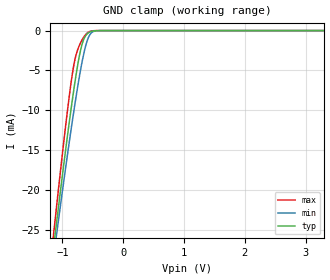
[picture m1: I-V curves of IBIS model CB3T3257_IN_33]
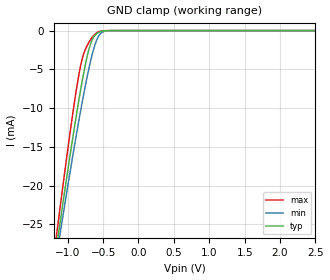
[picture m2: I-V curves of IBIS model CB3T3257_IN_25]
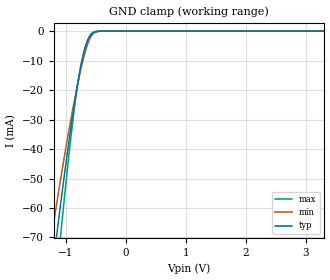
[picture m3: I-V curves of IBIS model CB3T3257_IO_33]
| TEXAS INSTRUMENTS INCORPORATED
| Standard Linear and Logic Group
| IBIS Model of SN74CB3T3257
| 3.3-V LOW-VOLTAGE 4-BIT 1-OF-2 FET MULTIPLEXER/DEMULTIPLEXER WITH 5-V-
| TOLERANT/LEVEL SHIFTER
| This file contains package information for the following:
|  TSSOP 16-pin (PW) package as [Component] CB3T3257_PW
|  TVSOP 16-pin (DGV) package as [Component] CB3T3257_DGV
| This device can be powered at the following Vccs:
|  3.3 volt Vcc
|  2.5 volt Vcc
| This file provides unique models under the [Model Selector] for each Vcc.
| For operation at a specific Vcc, select the appropriate model after each
| [Model Selector] keyword.
[IBIS Ver]   3.2
[Comment char]  |_char
[File Name]   sn74cb3t3257.ibs
[File Rev]   1.1 | a_die
[Date]   August 21, 2003
[Source]   Data created from TI-SPICE simulations at TI-SLL.
[Notes]   The following is an IBIS list for the CB3T3257.
   Please contact sllibis@ti.com with questions and
   comments concerning SLL IBIS models.
   - Non-monotonic data due to FET characteristics.
   - Power clamp data deleted as there is no power-clamp diode.
[Disclaimer] Property of Texas Instruments Incorporated.  Unauthorized
   reproduction and/or distribution is strictly prohibited.
   This product is protected under copyright law.
   Created  2003, (C) Copyright  2003, Texas Instruments
   Incorporated, All Rights Reserved
   UNLESS THERE IS A SIGNED, WRITTEN AGREEMENT TO THE
   CONTRARY, TEXAS INSTRUMENTS (TI) IS PROVIDING THE IBIS
   MODELS  AND WITHOUT ANY WARRANTY, EXPRESSED OR
   IMPLIED.  TI assumes no liability for:
   1) the accuracy of the IBIS models provided to your
   company;
   2) the proper functioning of these IBIS Models in your
   design or for any resulting applications; or
   3) infringement of patents, copyrights or intellectual
   property rights resulting from your use of these IBIS
   models.
   TI provides IBIS Models as a service to our customers.
   You and your company shall not distribute, sell or give
   these models to anyone else without prior written
   permission from TI.
   TI reserves the right to make changes to our products or
   to discontinue any semiconductor product or service
   without notice, and advises our customers to obtain the
   latest version of relevant information to verify, before
   placing orders, that the information being relied on is
   current.
   Please be aware that your receipt and use of the IBIS
   information provided shall serve as acceptance of these
   terms and conditions.  If you do not accept these terms,
   you should return or destroy the IBIS models and any
   other accompanying information immediately.
| Component CB3T3257_PW 16-pin TSSOP
[Component]   CB3T3257_PW
[Manufacturer]   Texas Instruments, Inc.
[Package]
|   typ   min   max
R_pkg   4.500e-02   3.800e-02   5.100e-02
L_pkg   2.593e-09   2.447e-09   3.080e-09
C_pkg   2.810e-13   2.430e-13   3.770e-13
[Pin]   signal_name   model_name   R_pin   L_pin   C_pin
1   S   CB3T3257_IN   4.000e-02   3.080e-09   3.770e-13
2   1B1   CB3T3257_IO   3.800e-02   2.458e-09   2.810e-13
3   1B2   CB3T3257_IO   5.100e-02   2.512e-09   2.550e-13
4   1A   CB3T3257_IO   5.100e-02   2.447e-09   2.430e-13
5   2B1   CB3T3257_IO   5.100e-02   2.447e-09   2.430e-13
6   2B2   CB3T3257_IO   5.100e-02   2.512e-09   2.550e-13
7   2A   CB3T3257_IO   3.800e-02   2.458e-09   2.810e-13
8   GND   GND   4.000e-02   3.080e-09   3.770e-13
9   3A   CB3T3257_IO   3.900e-02   2.832e-09   3.160e-13
10   3B2   CB3T3257_IO   3.800e-02   2.460e-09   2.790e-13
11   3B1   CB3T3257_IO   5.100e-02   2.512e-09   2.550e-13
12   4A   CB3T3257_IO   5.100e-02   2.447e-09   2.430e-13
13   4B2   CB3T3257_IO   5.100e-02   2.447e-09   2.430e-13
14   4B1   CB3T3257_IO   5.100e-02   2.512e-09   2.550e-13
15   NOE   CB3T3257_IN   3.800e-02   2.459e-09   2.790e-13
16   VCC   POWER   3.900e-02   2.832e-09   3.160e-13
| Component CB3T3257_DGV 16-pin TVSOP
[Component]   CB3T3257_DGV
[Manufacturer]   Texas Instruments, Inc.
[Package]
|   typ   min   max
R_pkg   3.900e-02   3.300e-02   4.500e-02
L_pkg   2.543e-09   2.320e-09   2.938e-09
C_pkg   3.860e-13   3.340e-13   4.490e-13
[Pin]   signal_name   model_name   R_pin   L_pin   C_pin
1   S   CB3T3257_IN   3.500e-02   2.907e-09   4.170e-13
2   1B1   CB3T3257_IO   4.200e-02   2.558e-09   4.460e-13
3   1B2   CB3T3257_IO   3.800e-02   2.341e-09   3.450e-13
4   1A   CB3T3257_IO   3.800e-02   2.320e-09   3.340e-13
5   2B1   CB3T3257_IO   3.900e-02   2.322e-09   3.340e-13
6   2B2   CB3T3257_IO   3.800e-02   2.353e-09   3.420e-13
7   2A   CB3T3257_IO   4.000e-02   2.536e-09   4.410e-13
8   GND   GND   3.300e-02   2.897e-09   4.180e-13
9   3A   CB3T3257_IO   3.500e-02   2.927e-09   4.190e-13
10   3B2   CB3T3257_IO   4.500e-02   2.632e-09   4.490e-13
11   3B1   CB3T3257_IO   3.900e-02   2.368e-09   3.470e-13
12   4A   CB3T3257_IO   3.900e-02   2.330e-09   3.350e-13
13   4B2   CB3T3257_IO   3.900e-02   2.320e-09   3.350e-13
14   4B1   CB3T3257_IO   3.900e-02   2.361e-09   3.450e-13
15   NOE   CB3T3257_IN   4.100e-02   2.573e-09   4.460e-13
16   VCC   POWER   3.500e-02   2.938e-09   4.200e-13
[Series Switch Groups]
| Function Group States
On  1 /   | 1A->1B1 NOE LOW S LOW
   | 2A->2B1 NOE LOW S LOW
   | 3A->3B1 NOE LOW S LOW
   | 4A->4B1 NOE LOW S LOW
On  2 /   | 1A->1B2 NOE LOW S HIGH
   | 2A->2B2 NOE LOW S HIGH
   | 3A->3B2 NOE LOW S HIGH
   | 4A->4B2 NOE LOW S HIGH
Off 1 2 /   | NOE HIGH
[Series Pin Mapping]   pin_2   model_name   function_table_group
4   2   CB3T3257_IO_33_S   1
| 4   2   CB3T3257_IO_25_S   1
4   3   CB3T3257_IO_33_S   2
| 4   3   CB3T3257_IO_25_S   2
7   5   CB3T3257_IO_33_S   1
| 7   5   CB3T3257_IO_25_S   1
7   6   CB3T3257_IO_33_S   2
| 7   6   CB3T3257_IO_25_S   2
9   11   CB3T3257_IO_33_S   1
| 9   11   CB3T3257_IO_25_S   1
9   10   CB3T3257_IO_33_S   2
| 9   10   CB3T3257_IO_25_S   2
12   14   CB3T3257_IO_33_S   1
| 12   14   CB3T3257_IO_25_S   1
12   13   CB3T3257_IO_33_S   2
| 12   13   CB3T3257_IO_25_S   2
| Model CB3T3257_IN
[Model Selector]   CB3T3257_IN
CB3T3257_IN_33   3.3 volt Vcc
CB3T3257_IN_25   2.5 volt Vcc
| Model CB3T3257_IO
[Model Selector]   CB3T3257_IO
CB3T3257_IO_33   3.3 volt Vcc
CB3T3257_IO_25   2.5 volt Vcc
| Model CB3T3257_IO_S
[Model Selector]   CB3T3257_IO_S
CB3T3257_IO_33_S   3.3 volt Vcc_S
CB3T3257_IO_25_S   2.5 volt Vcc_S
[Model]   CB3T3257_IO_33_S
Model_type  Series_switch
| variable   typ   min   max
C_comp   0   0   0
[Temperature Range]   40   100   -40
| Ambient temperature   25   85   -40
[Voltage range]   3.3   3   3.6
[On]
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[Off]
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[Model]   CB3T3257_IO_25_S
Model_type  Series_switch
| variable   typ   min   max
C_comp   0   0   0
[Temperature Range]   40   100   -40
| Ambient temperature   25   85   -40
[Voltage range]   2.5   2.3   2.7
[On]
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[Off]
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| Models and submodels in the file (6): CB3T3257_IN_33 (Input), CB3T3257_IN_25 (Input), CB3T3257_IO_33_S (Series_switch), CB3T3257_IO_33 (Terminator), CB3T3257_IO_25_S (Series_switch), CB3T3257_IO_25 (Terminator)
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[Model]   CB3T3257_IN_33
Model_type  Input
Vinl=0.8
Vinh=2.0
| variable   typ   min   max
C_comp   2.59pF   2.02pF   3.28pF
[Temperature Range]   40   100   -40
| Ambient temperature   25   85   -40
[Voltage range]   3.3   3   3.6
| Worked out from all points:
|   GND clamp passes 1 mA (typ) near -0.64 V on its own axis
[GND Clamp]
| CB3T3257_IN_33
|   Voltage   I(typ)   I(min)   I(max)
-5.5V     -338.9mA   -314.3mA   -369mA
-1.14V    -26.82mA   -28.07mA   -25.13mA
-1.105V   -24.61mA   -26.05mA   -22.65mA
-1.075V   -22.73mA   -24.34mA   -20.55mA
-915mV    -13.07mA   -15.45mA   -9.893mA
-860mV    -9.954mA   -12.53mA   -6.658mA
-805mV    -7.019mA   -9.733mA   -4.027mA
-730mV    -3.528mA   -6.174mA   -2.02mA
-665mV    -1.428mA   -3.486mA   -1.009mA
-585mV    -362.1uA   -1.111mA   -263.9uA
-510mV    -78.77uA   -204.1uA   -38.82uA
3.3V      76.2pA     212.8pA    43.07pA
[Model]   CB3T3257_IN_25
Model_type  Input
Vinl=0.7
Vinh=1.7
| variable   typ   min   max
C_comp   2.66pF   2.08pF   3.27pF
[Temperature Range]   40   100   -40
| Ambient temperature   25   85   -40
[Voltage range]   2.5   2.3   2.7
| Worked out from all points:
|   GND clamp passes 1 mA (typ) near -0.64 V on its own axis
[GND Clamp]
| CB3T3257_IN_25
|   Voltage   I(typ)   I(min)   I(max)
-5.5V     -338.9mA   -314.3mA   -369mA
-1.17V    -28.73mA   -29.82mA   -27.27mA
-1.13V    -26.19mA   -27.5mA    -24.42mA
-1.095V   -23.98mA   -25.48mA   -21.95mA
-925mV    -13.65mA   -15.98mA   -10.52mA
-825mV    -8.06mA    -10.74mA   -4.88mA
-775mV    -5.531mA   -8.266mA   -3.027mA
-700mV    -2.416mA   -4.874mA   -1.51mA
-590mV    -396.4uA   -1.217mA   -293.2uA
-515mV    -88.16uA   -231.8uA   -44.89uA
-395mV    -4.232uA   -9.445uA   -775nA
2.5V      57.25pA    176.8pA    32.61pA
[Model]   CB3T3257_IO_33
Model_type  Terminator
| variable   typ   min   max
C_comp   3.99pF   3.07pF   5.16pF
| C_tri-state   3.99pF   3.07pF   5.16pF
[Temperature Range]   40   100   -40
| Ambient temperature   25   85   -40
[Voltage range]   3.3   3   3.6
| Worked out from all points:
|   GND clamp passes 1 mA (typ) near -0.56 V on its own axis
[GND Clamp]
| CB3T3257_IO_33
|   Voltage   I(typ)   I(min)   I(max)
-5.5V     -1.008A    -841.1mA   -1.184A
-1.24V    -84.16mA   -70.17mA   -102.1mA
-1.195V   -76.47mA   -64.15mA   -92.27mA
-1.15V    -68.95mA   -58.26mA   -82.61mA
-1.09V    -59.17mA   -50.61mA   -70.01mA
-1.07V    -55.99mA   -48.11mA   -65.89mA
-890mV    -29.27mA   -27.07mA   -31.52mA
-790mV    -16.49mA   -16.78mA   -16.36mA
-675mV    -5.462mA   -6.985mA   -5.356mA
-550mV    -740.6uA   -1.02mA    -478.1uA
-325mV    -2.166uA   -4.071uA   -187.7nA
3.3V      246.4pA    10.98nA    81.93pA
